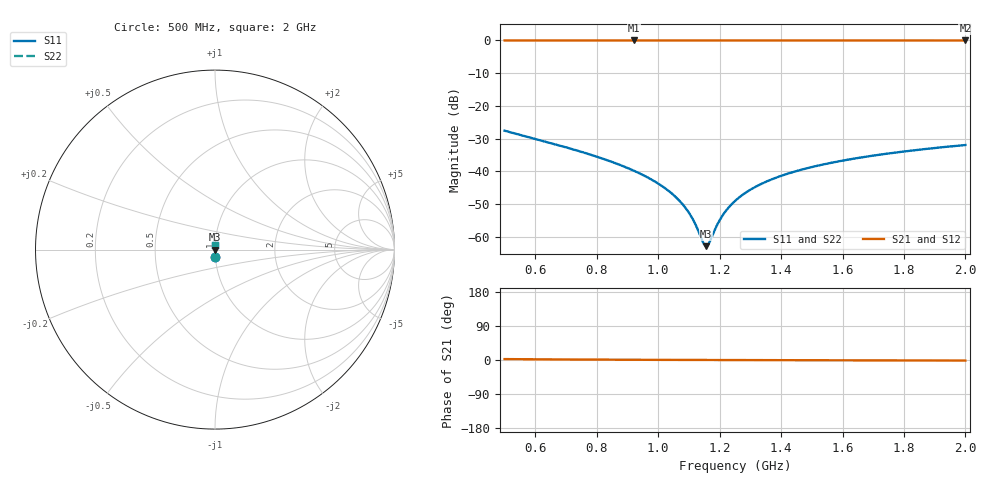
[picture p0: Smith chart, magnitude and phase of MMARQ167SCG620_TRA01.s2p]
! MMARQ167SCG620_TRA01  S-PARAMETER MODEL  ( General Type )
! Model Generated by TAIYO YUDEN Corporation (http://www.ty-top.com)
! Version 1.0
! TAIYO YUDEN Control No. 160201
! Copyright(c) 2016 TAIYO YUDEN CO.,LTD. All Rights Reserved.
! Product Description (link to TY-COMPAS)
! https://ds.yuden.co.jp/TYCOMPAS/or/detail?pn=MMARQ167SCG620JTRA01&u=M
! Products Name : Multilayer Ceramic Capacitors
! Characteristics :
!  Capacitance : 62 pF , Rated Voltage : 250V , TCC : CG / C0G
!  Case Size : 1.6 x 0.8 / 0.063 x 0.031 [mm/inch] , Thickness : 0.7 / 0.028 [mm/inch]
!  (Conditions: Temperature = 25 degC , DC Bias Current/Voltage = 0A / 0V)
! External Node Assignments :
!  1  o---| |---o  2
! GND o---------o GND
! Frequency Range : 500MHz  -  2000MHz  [ 401 STEP ]
# MHz S RI R 50
! Freq[MHz].  S11 Real  S11 Imag  S21 Real  S21 Imag  S12 Real  S12 Imag  S22 Real  S22 Imag
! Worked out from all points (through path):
!   401 points, 500 MHz to 2 GHz, reference 50 ohm
!   highest |S21| = -0.01 dB at 920 MHz (marker M1); lowest = 0.0 dB at 2 GHz (marker M2)
!   lowest |S11| = -62.9 dB at 1.156 GHz (marker M3), VSWR 1.00, Z = 50.1 - j0.00171 ohm
!   |S11| at or under -10 dB: start of sweep to end of sweep
!   |S22| runs from -62.9 to -27.6 dB; largest |S21 - S12| = 0
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500  0.0022 -0.0416  0.9978 0.0416  0.9978 0.0416  0.0022 -0.0416
751.25  0.000896 -0.0197  0.9991 0.0197  0.9991 0.0197  0.000896 -0.0197
845  0.000746 -0.0141  0.9993 0.0141  0.9993 0.0141  0.000746 -0.0141
920  0.000687 -0.0102  0.9993 0.0102  0.9993 0.0102  0.000687 -0.0102
1002.5  0.000666 -0.00634  0.9993 0.00634  0.9993 0.00634  0.000666 -0.00634
1051.25  0.000671 -0.00423  0.9993 0.00423  0.9993 0.00423  0.000671 -0.00423
1088.75  0.000682 -0.00267  0.9993 0.00267  0.9993 0.00267  0.000682 -0.00267
1115  0.000693 -0.00162  0.9993 0.00162  0.9993 0.00162  0.000693 -0.00162
1145  0.000709 -0.000448  0.9993 0.000448  0.9993 0.000448  0.000709 -0.000448
1156.25  0.000715 -1.71e-05  0.9993 1.71e-05  0.9993 1.71e-05  0.000715 -1.71e-05
1167.5  0.000722 0.00041  0.9993 -0.00041  0.9993 -0.00041  0.000722 0.00041
1190  0.000737 0.00125  0.9993 -0.00125  0.9993 -0.00125  0.000737 0.00125
1208.75  0.000751 0.00194  0.9992 -0.00194  0.9992 -0.00194  0.000751 0.00194
1227.5  0.000766 0.00262  0.9992 -0.00262  0.9992 -0.00262  0.000766 0.00262
1250  0.000785 0.00342  0.9992 -0.00342  0.9992 -0.00342  0.000785 0.00342
1295  0.000827 0.00498  0.9992 -0.00498  0.9992 -0.00498  0.000827 0.00498
1351.25  0.000886 0.00687  0.9991 -0.00687  0.9991 -0.00687  0.000886 0.00687
1418.75  0.000965 0.00904  0.999 -0.00904  0.999 -0.00904  0.000965 0.00904
1501.25  0.00107 0.0116  0.9989 -0.0116  0.9989 -0.0116  0.00107 0.0116
1613.75  0.00124 0.0149  0.9988 -0.0149  0.9988 -0.0149  0.00124 0.0149
1752.5  0.00146 0.0187  0.9985 -0.0187  0.9985 -0.0187  0.00146 0.0187
2000  0.00191 0.0251  0.9981 -0.0251  0.9981 -0.0251  0.00191 0.0251
